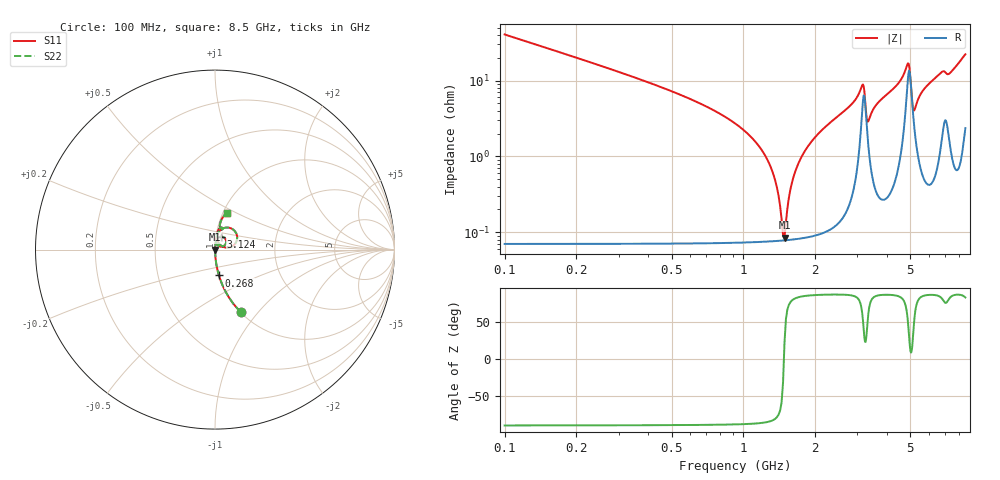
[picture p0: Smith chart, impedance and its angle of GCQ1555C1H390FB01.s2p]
!Murata Part Number: GCQ1555C1H390FB01
!These Parameters are Measured in Series Mode Connection
!Data Generated on Jan 08, 2026
!  o--ll--o
!Port1  Port2
!  o------o
!Operation Temp=25[degC], DC Bias Voltage=0[V]
!Freq. Start=100[MHz] Stop=9[GHz] 401[Steps]
# Hz S RI R 50
!Freq.(Hz) S11(Real) S11(Imag) S21(Real) S21(Imag) S12(Real) S12(Imag) S22(Real) S22(Imag)
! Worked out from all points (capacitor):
!   401 points, 100 MHz to 8.5 GHz, reference 50 ohm
!   read as one part in series: C = 39 pF near 142 MHz
!   lowest |Z| = 84.6 mohm at 1.486 GHz (marker M1)
!   series resonance near 1.478 GHz, so ESL is about 300 pH
!   S11 on the Smith chart (normalised r, x): 100 MHz: 1.00, -0.81; 268 MHz: 1.00, -0.29; 3.124 GHz: 1.06, +0.15; 8.5 GHz: 1.05, +0.44
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1e8  0.1421 -0.3483  0.8579 0.3483  0.8579 0.3483  0.1421 -0.3483
2.68e8  0.0219 -0.144  0.9781 0.144  0.9781 0.144  0.0219 -0.144
1.192e9  0.000893 -0.0121  0.9991 0.0121  0.9991 0.0121  0.000893 -0.0121
1.339e9  0.000791 -0.00556  0.9992 0.00556  0.9992 0.00556  0.000791 -0.00556
1.444e9  0.000775 -0.0013  0.9992 0.0013  0.9992 0.0013  0.000775 -0.0013
1.486e9  0.00078 0.000326  0.9992 -0.000326  0.9992 -0.000326  0.00078 0.000326
1.507e9  0.000784 0.00112  0.9992 -0.00112  0.9992 -0.00112  0.000784 0.00112
1.633e9  0.000837 0.00573  0.9992 -0.00573  0.9992 -0.00573  0.000837 0.00573
1.843e9  0.00102 0.0129  0.999 -0.0129  0.999 -0.0129  0.00102 0.0129
2.914e9  0.00691 0.053  0.9931 -0.053  0.9931 -0.053  0.00691 0.053
3.124e9  0.0347 0.0724  0.9653 -0.0724  0.9653 -0.0724  0.0347 0.0724
3.187e9  0.0625 0.0493  0.9375 -0.0493  0.9375 -0.0493  0.0625 0.0493
3.292e9  0.0225 0.0189  0.9775 -0.0189  0.9775 -0.0189  0.0225 0.0189
3.334e9  0.0143 0.0249  0.9857 -0.0249  0.9857 -0.0249  0.0143 0.0249
3.628e9  0.00558 0.0489  0.9944 -0.0489  0.9944 -0.0489  0.00558 0.0489
4.3e9  0.011 0.0801  0.989 -0.0801  0.989 -0.0801  0.011 0.0801
4.888e9  0.1103 0.1035  0.8897 -0.1035  0.8897 -0.1035  0.1103 0.1035
5.182e9  0.0262 0.0293  0.9738 -0.0293  0.9738 -0.0293  0.0262 0.0293
5.707e9  0.0108 0.076  0.9892 -0.076  0.9892 -0.076  0.0108 0.076
6.736e9  0.0299 0.1219  0.9701 -0.1219  0.9701 -0.1219  0.0299 0.1219
7.114e9  0.0388 0.1121  0.9612 -0.1121  0.9612 -0.1121  0.0388 0.1121
8.5e9  0.0668 0.2018  0.9332 -0.2018  0.9332 -0.2018  0.0668 0.2018
